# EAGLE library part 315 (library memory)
MEMORY
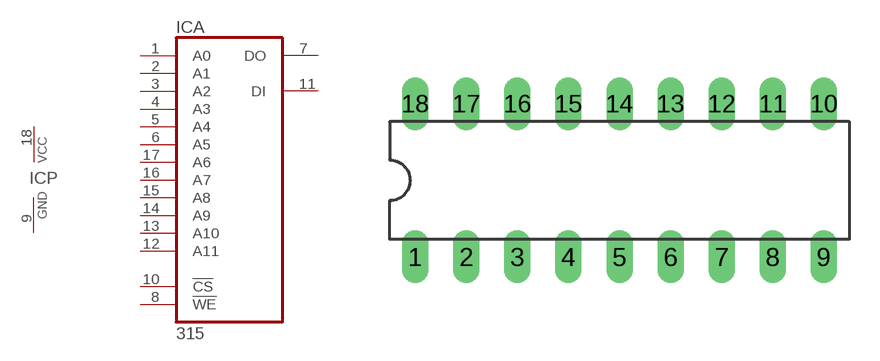
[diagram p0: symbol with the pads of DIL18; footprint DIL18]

Designator prefix IC; gates A=315 P=PWRN

## 315  [DIL18]
1  A:A0  in
2  A:A1  in
3  A:A2  in
4  A:A3  in
5  A:A4  in
6  A:A5  in
7  A:DO  hiz
8  A:!WE  in
9  P:GND  pwr
10  A:!CS  in
11  A:DI  in
12  A:A11  in
13  A:A10  in
14  A:A9  in
15  A:A8  in
16  A:A7  in
17  A:A6  in
18  P:VCC  pwr

## Footprint DIL18 (pad centres in mm)
Dual In Line Package
drill 0.813 long: 1 -10.16,-3.81; 2 -7.62,-3.81; 3 -5.08,-3.81; 4 -2.54,-3.81; 5 0,-3.81; 6 2.54,-3.81; 7 5.08,-3.81; 8 7.62,-3.81; 9 10.16,-3.81; 10 10.16,3.81; 11 7.62,3.81; 12 5.08,3.81; 13 2.54,3.81; 14 0,3.81; 15 -2.54,3.81; 16 -5.08,3.81; 17 -7.62,3.81; 18 -10.16,3.81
